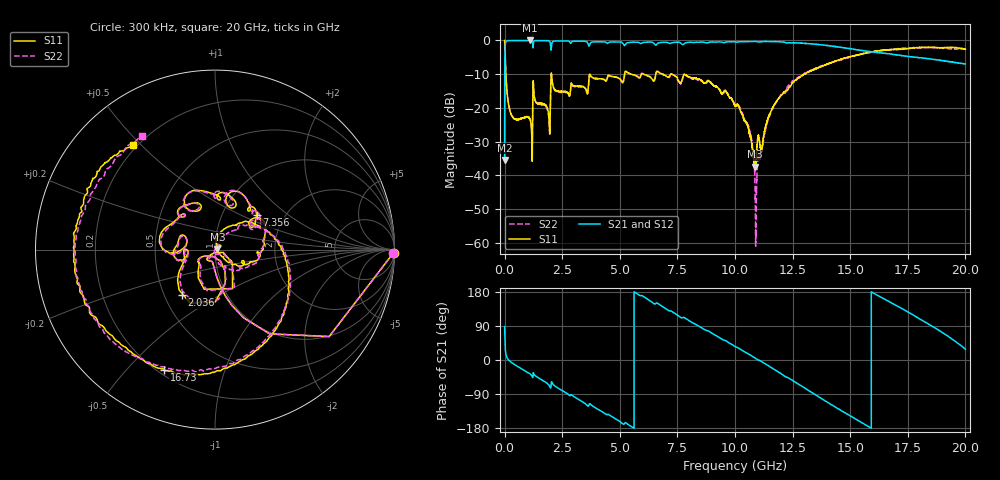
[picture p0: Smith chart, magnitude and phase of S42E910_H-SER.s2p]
!{S42E910}
!Johanson Technology Inc.
!www.johansontechnology.com
!Test Board Conditions:
!Substrate Type  RO4350B
!Substrate Thickness  50 mil
!Substrate Dk  3.66
!TL Type: GCPW
!TL Trace Width  60 mil
!TL Gap  10 mil
!Electrode orientation  Horizontal
!DUT TOPOLOGY	SERIES
!Mounting Pad LxW  14x55 mil
! Created Wed Nov 25 22:28:41 2020
# khz S ma R 50
! 2 Port Network Data from SP1.SP block
! freq  magS11  angS11  magS21  angS21  magS12  angS12  magS22  angS22
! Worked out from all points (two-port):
!   20001 points, 300 kHz to 20 GHz, reference 50 ohm
!   highest |S21| = -0.03 dB at 1.096 GHz (marker M1); lowest = -35.5 dB at 300 kHz (marker M2)
!   |S21| within 3 dB of the highest: 17.76 MHz to 15.53 GHz (15.51 GHz wide, 200 % of centre); 15.53636 GHz to 15.53751 GHz (1.151 MHz wide, 0.00741 % of centre)
!   lowest |S11| = -37.4 dB at 10.87 GHz (marker M3), VSWR 1.03, Z = 51.3 + j0.365 ohm
!   |S11| at or under -10 dB: 53.55 MHz to 2.02 GHz (1.966 GHz wide, 190 % of centre); 2.035 GHz to 3.686 GHz (1.65 GHz wide, 57.7 % of centre); 7.255 GHz to 13 GHz (5.746 GHz wide, 56.7 % of centre)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
!   |S22| runs from -60.9 to 0.0 dB; largest |S21 - S12| = 0.02
!   S11 on the Smith chart (normalised r, x): 300 kHz: open; 2.036 GHz: 0.61, -0.34; 7.356 GHz: 1.45, +0.62; 16.73 GHz: 0.23, -0.64; 20 GHz: 0.19, +0.48
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300  0.9951 -1.0  0.01688 88.0  0.01691 89.1  0.9944 -1.1
116300  0.1575 -85.8  0.9857 4.8  0.986 4.8  0.1584 -85.8
356300  0.07264 -101.0  0.9954 -9.0  0.9958 -9.0  0.07332 -99.7
1096300  0.0684 -130.7  0.997 -36.4  0.9958 -36.4  0.06988 -123.1
1317300  0.1302 -133.6  0.9876 -40.8  0.9867 -40.8  0.1328 -127.0
1885300  0.09149 -151.2  0.9888 -63.6  0.989 -63.6  0.08691 -150.4
2036300  0.3141 -126.4  0.8348 -57.3  0.8348 -57.3  0.3058 -123.2
3334300  0.2092 160.2  0.9715 -108.4  0.9714 -108.4  0.2061 162.8
4990300  0.2711 109.0  0.9487 -161.7  0.9486 -161.8  0.2713 110.4
6667300  0.3407 61.5  0.9122 148.4  0.909 148.3  0.3431 63.0
7356300  0.3023 40.0  0.9354 124.1  0.9344 124.2  0.3052 32.5
8555300  0.2531 -4.0  0.9444 84.8  0.943 84.9  0.2489 -5.5
1.00003e7  0.1071 -37.1  0.9518 35.6  0.9522 35.6  0.1084 -58.3
1.06293e7  0.04149 -44.1  0.9637 14.2  0.9625 14.2  0.04537 -86.0
1.08703e7  0.0135 15.3  0.9654 5.2  0.9663 5.2  0.007305 -107.2
1.16663e7  0.1047 71.8  0.9614 -23.5  0.9606 -23.4  0.1029 54.9
1.33343e7  0.3597 4.0  0.8861 -85.7  0.8871 -85.5  0.3637 5.1
1.49933e7  0.5724 -56.7  0.7535 -147.1  0.7515 -147.4  0.5662 -57.9
1.66673e7  0.7226 -110.6  0.6352 155.0  0.6199 154.9  0.7265 -118.8
1.67303e7  0.7269 -112.9  0.6281 152.8  0.6144 153.0  0.7281 -120.6
1.83023e7  0.7848 -173.8  0.5395 98.0  0.5398 98.8  0.7811 -165.4
2e7  0.7382 127.9  0.4477 28.6  0.4512 29.4  0.7494 122.7
